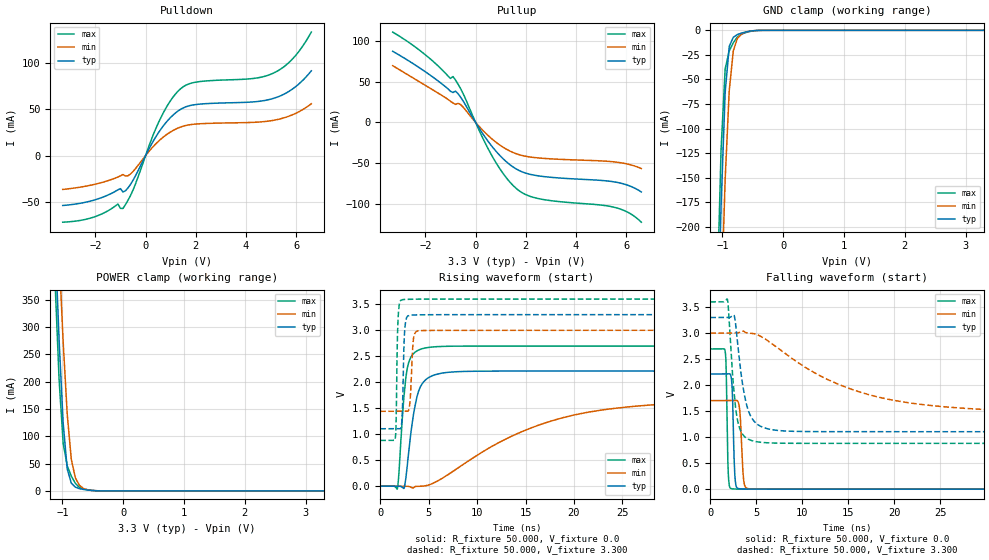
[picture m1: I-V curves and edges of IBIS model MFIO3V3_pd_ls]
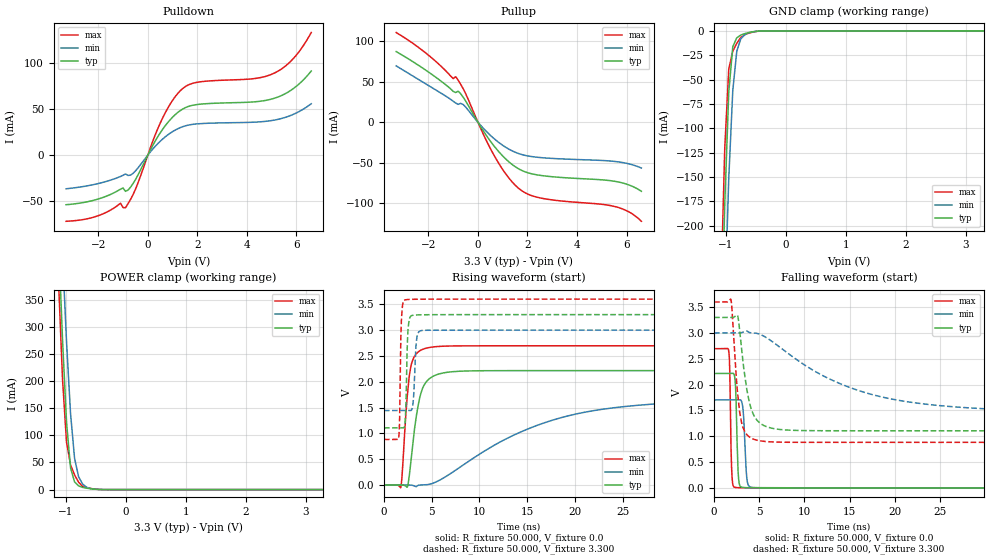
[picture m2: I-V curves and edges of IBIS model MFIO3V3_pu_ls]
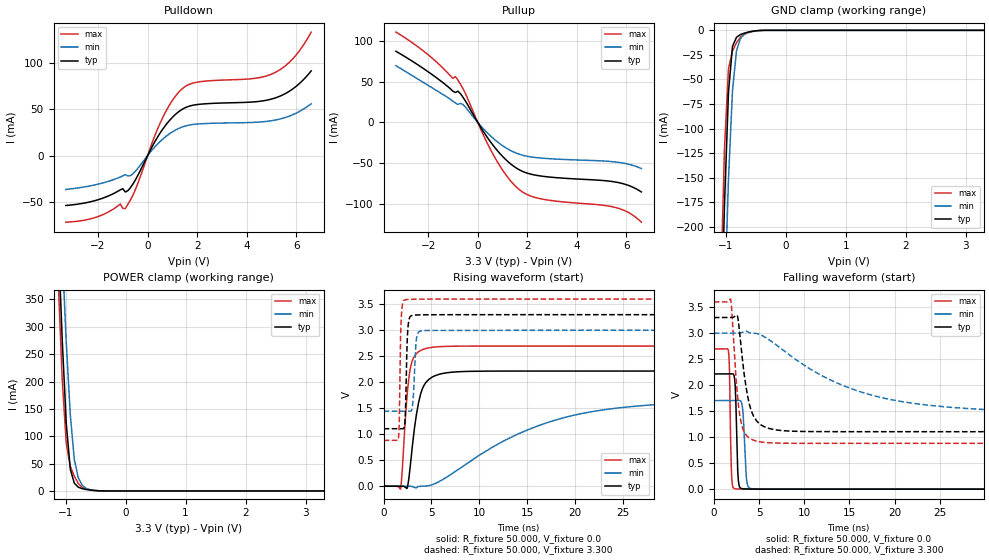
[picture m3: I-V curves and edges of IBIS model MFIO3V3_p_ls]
| IBIS file lpc55s0x_jbd64.ibs
[IBIS Ver]   5.0
[File name]   lpc55s0x_jbd64.ibs
[File Rev]   1.0
[Date]   August 08,2020
[Notes]   Rev History
|   1.0  initial release
[Disclaimer]   The model given below represents a 64-pin package.
[Copyright]   Copyright NXP 2020
[Component] lpc55s0x
[Manufacturer] NXP
[Package]
|   typ   min   max
R_pkg   0.19617   0.1259   0.24257
L_pkg   3.452e-9   2.657e-9   4.299e-9
C_pkg   5.434e-13   4.645e-13   6.669e-13
[Pin]   Signal_name   model_name   R_pin   L_pin   C_pin
32   VBAT_DCDC   POWER   NA   NA   NA
33   VBAT_PMU   POWER   NA   NA   NA
9   VDDA   POWER   NA   NA   NA
8   VDDE   POWER   NA   NA   NA
16   VDDE   POWER   NA   NA   NA
28   VDDE   POWER   NA   NA   NA
43   VDDE   POWER   NA   NA   NA
56   VDDE   POWER   NA   NA   NA
24   VDD_PMU   POWER   NA   NA   NA
10   VREFP   POWER   NA   NA   NA
29   FB   NC   0.21382   3.234e-9   5.594e-13
31   LX   NC   0.1259   2.657e-9   6.669e-13
36   P0_0   gpio3v3   0.18104   3.304e-9   5.312e-13
2   P0_1   gpio3v3   0.20833   3.785e-9   5.955e-13
54   P0_2   gpio3v3   0.19647   3.418e-9   5.268e-13
55   P0_3   gpio3v3   0.2007   3.265e-9   5.08e-13
57   P0_4   gpio3v3   0.20065   3.267e-9   5.147e-13
58   P0_5   gpio3v3   0.20039   3.463e-9   5.189e-13
59   P0_6   gpio3v3   0.20514   3.553e-9   5.526e-13
1   P0_7   gpio3v3   0.22402   4.088e-9   5.574e-13
17   P0_8   gpio3v3   0.21685   3.93e-9   5.333e-13
37   P0_9   gpio3v3   0.17288   3.178e-9   5.157e-13
13   P0_10   gpio3v3   0.18436   3.37e-9   5.571e-13
6   P0_11   gpio3v3   0.17442   3.19e-9   5.137e-13
5   P0_12   gpio3v3   0.18127   3.344e-9   5.397e-13
46   P0_13   iicgpio3v3   0.18768   3.399e-9   5.469e-13
47   P0_14   iicgpio3v3   0.19847   3.574e-9   5.659e-13
14   P0_15   gpio3v3   0.19509   3.491e-9   5.923e-13
7   P0_16   gpio3v3   0.17362   2.955e-9   4.961e-13
38   P0_18   gpio3v3   0.16738   3.09e-9   4.89e-13
60   P0_19   gpio3v3   0.21213   3.67e-9   5.623e-13
48   P0_20   gpio3v3   0.20914   3.854e-9   5.212e-13
49   P0_21   gpio3v3   0.22547   4.105e-9   5.559e-13
51   P0_22   gpio3v3   0.20602   3.668e-9   5.785e-13
12   P0_23   gpio3v3   0.17829   3.098e-9   5.305e-13
45   P0_24   gpio3v3   0.17877   3.257e-9   5.192e-13
52   P0_25   gpio3v3   0.2005   3.571e-9   5.586e-13
40   P0_26   gpio3v3   0.16383   2.973e-9   4.854e-13
18   P0_27   gpio3v3   0.20727   3.705e-9   5.696e-13
44   P0_28   gpio3v3   0.17962   3.062e-9   4.989e-13
61   P0_29   gpio3v3   0.21833   3.792e-9   5.854e-13
63   P0_30   gpio3v3   0.24257   4.299e-9   6.149e-13
15   P0_31   gpio3v3   0.21237   3.493e-9   6.058e-13
4   P1_0   gpio3v3   0.19044   3.496e-9   5.532e-13
39   P1_1   gpio3v3   0.16532   3.035e-9   4.645e-13
41   P1_2   gpio3v3   0.16584   2.976e-9   4.885e-13
42   P1_3   gpio3v3   0.17391   2.979e-9   4.668e-13
64   P1_4   gpio3v3   0.21758   3.972e-9   5.207e-13
22   P1_5   gpio3v3   0.19606   3.418e-9   5.2e-13
3   P1_9   gpio3v3   0.20144   3.654e-9   5.698e-13
25   P1_10   gpio3v3   0.20199   3.169e-9   5.208e-13
62   P1_11   gpio3v3   0.22784   3.919e-9   6.247e-13
21   P1_21   gpio3v3   0.19848   3.493e-9   5.331e-13
26   P1_22   gpio3v3   0.19791   3.34e-9   5.122e-13
27   P1_23   gpio3v3   0.20351   3.333e-9   5.169e-13
50   P1_25   gpio3v3   0.21369   3.798e-9   6.012e-13
53   P1_29   gpio3v3   0.19707   3.477e-9   5.49e-13
23   RESETN   gpio3v3   0.19717   3.324e-9   5.017e-13
35   XTAL32K_N   NC   0.18989   3.359e-9   5.665e-13
34   XTAL32K_P   NC   0.2095   3.368e-9   5.834e-13
19   XTAL32M_N   NC   0.20829   3.687e-9   5.553e-13
20   XTAL32M_P   NC   0.202   3.586e-9   5.404e-13
65   VSS   GND   NA   NA   NA
11   VSSA   GND   NA   NA   NA
30   VSS_DCDC   GND   NA   NA   NA
|   Model Selector
[Model Selector] gpio3v3
MFIO3V3_pd_hs  EPUN=1 EPD=1 EHS=1
MFIO3V3_pd_ls  EPUN=1 EPD=1 EHS=0
MFIO3V3_pu_hs  EPUN=0 EPD=0 EHS=1
MFIO3V3_pu_ls  EPUN=0 EPD=0 EHS=0
MFIO3V3_p_hs  EPUN=1 EPD=0 EHS=1
MFIO3V3_p_ls  EPUN=1 EPD=0 EHS=0
MFIO3V3_r_hs  EPUN=0 EPD=1 EHS=1
MFIO3V3_r_ls  EPUN=0 EPD=1 EHS=0
[Model Selector] iicgpio3v3
IIC3V3_pd_hs  EGP=1 EPUN=1 EPD=1 EHS=1
IIC3V3_pd_ls  EGP=1 EPUN=1 EPD=1 EHS=0
IIC3V3_p_hs  EGP=1 EPUN=1 EPD=0 EHS=1
IIC3V3_p_ls  EGP=1 EPUN=1 EPD=0 EHS=0
IIC3V3_pu_hs  EGP=1 EPUN=0 EPD=0 EHS=1
IIC3V3_pu_ls  EGP=1 EPUN=0 EPD=0 EHS=0
IIC3V3_r_hs  EGP=1 EPUN=0 EPD=1 EHS=1
IIC3V3_r_ls  EGP=1 EPUN=0 EPD=1 EHS=0
IIC3V3_pd_iic_hs  EGP=0 ECS=0 EPUN=1 EPD=1
IIC3V3_p_iic_hs  EGP=0 ECS=0 EPUN=1 EPD=0
IIC3V3_pu_iic_hs  EGP=0 ECS=0 EPUN=0 EPD=0
IIC3V3_r_iic_hs  EGP=0 ECS=0 EPUN=0 EPD=1
IIC3V3_pd_iic_pu_hs  EGP=0 ECS=1 EPUN=1 EPD=1  SSEL=1
IIC3V3_p_iic_pu_hs  EGP=0 ECS=1 EPUN=1 EPD=0  SSEL=1
IIC3V3_pu_iic_pu_hs  EGP=0 ECS=1 EPUN=0 EPD=0  SSEL=1
IIC3V3_r_iic_pu_hs  EGP=0 ECS=1 EPUN=0 EPD=1  SSEL=1
| Models and submodels in the file (24): MFIO3V3_pd_hs (I/O), MFIO3V3_pd_ls (I/O), MFIO3V3_pu_hs (I/O), MFIO3V3_pu_ls (I/O), MFIO3V3_p_hs (I/O), MFIO3V3_p_ls (I/O), MFIO3V3_r_hs (I/O), MFIO3V3_r_ls (I/O), IIC3V3_pd_hs (I/O), IIC3V3_pd_ls (I/O), IIC3V3_p_hs (I/O), IIC3V3_p_ls (I/O), IIC3V3_pu_hs (I/O), IIC3V3_pu_ls (I/O), IIC3V3_r_hs (I/O), IIC3V3_r_ls (I/O), IIC3V3_pd_iic_hs (I/O_open_drain), IIC3V3_p_iic_hs (I/O_open_drain), IIC3V3_pu_iic_hs (I/O_open_drain), IIC3V3_r_iic_hs (I/O_open_drain), IIC3V3_pd_iic_pu_hs (I/O_open_drain), IIC3V3_p_iic_pu_hs (I/O_open_drain), IIC3V3_pu_iic_pu_hs (I/O_open_drain), IIC3V3_r_iic_pu_hs (I/O_open_drain)
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|   Model MFIO3V3_pd_ls
[Model] MFIO3V3_pd_ls
Model_type I/O
Polarity   Non-Inverting
Enable   Active-Low
Vinl =  0.990V
Vinh =  2.310V
Vmeas =  1.650V
Cref =  0.0F
Rref =  100.000
Vref =  0.0V
C_comp   1.906pF   1.877pF   1.925pF
C_comp_pullup   1.141pF   1.113pF   1.145pF
C_comp_pulldown   0.641pF   0.601pF   0.647pF
[Model Spec]
Vinh   2.310V   2.100V   2.520V
Vinl   0.990V   0.900V   1.080V
Vmeas   1.650V   1.500V   1.800V
Vref   0.0V   0.0V   0.0V
Cref   0.0F   0.0F   0.0F
Rref   100.000   100.000   100.000
[Temperature Range]   25.000   0.125k   -40.000
[Voltage Range]   3.300V   3.000V   3.600V
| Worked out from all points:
|   slope of the pulldown table from 0 to 0.495 V, typ, clamps not added: 20.7 ohm
|   slope of the pullup table from 0 to 0.495 V, typ, clamps not added: 21.4 ohm
|   GND clamp passes 1 mA (typ) near -0.56 V on its own axis
|   POWER clamp passes 1 mA (typ) near -0.53 V on its own axis
|   rising waveform, R_fixture 50.000, V_fixture 0.0: 20-80 % time 1.05ns typ, 11.9ns min, 670ps max; typ from 0 V to 2.21 V
|   rising waveform, R_fixture 50.000, V_fixture 3.300: 20-80 % time 176ps typ, 234ps min, 146ps max; typ from 1.1 V to 3.3 V
|   falling waveform, R_fixture 50.000, V_fixture 0.0: 20-80 % time 203ps typ, 279ps min, 162ps max; typ from 2.21 V to 0 V
|   falling waveform, R_fixture 50.000, V_fixture 3.300: 20-80 % time 1.13ns typ, 11.2ns min, 744ps max; typ from 3.3 V to 1.1 V
[Pulldown]
|Voltage   I(typ)   I(min)   I(max)
-3.3V     -53.7mA    -36.43mA   -71.67mA
-2.1V     -48.29mA   -31.37mA   -66.51mA
-1.1V     -36.82mA   -23.05mA   -52.1mA
-900mV    -39.2mA    -20.39mA   -56.91mA
-600mV    -30.96mA   -19.83mA   -42.97mA
600mV     28.07mA    17.5mA     40.4mA
1V        41.17mA    25.53mA    59.41mA
1.4V      49.87mA    30.79mA    72.04mA
2V        54.93mA    33.94mA    79.03mA
5V        60.84mA    37.53mA    87.68mA
5.9V      72.62mA    44.52mA    105.4mA
6.6V      91.19mA    55.78mA    132.9mA
[Pullup]
|Voltage   I(typ)   I(min)   I(max)
-3.3V     87.16mA    69.54mA    110.7mA
-2.1V     64.12mA    47.22mA    85.31mA
-1V       38.1mA     25.85mA    53.88mA
-900mV    36.64mA    23.75mA    56.16mA
-800mV    38.25mA    22.02mA    51.93mA
-600mV    31.06mA    21.93mA    41.58mA
700mV     -31.25mA   -21.55mA   -43.56mA
1.2V      -47.6mA    -32.42mA   -66.97mA
1.7V      -58.52mA   -39.3mA    -83.05mA
2.6V      -66.01mA   -43.88mA   -94.06mA
5.6V      -73.4mA    -48.74mA   -104.7mA
6.6V      -85.32mA   -56.6mA    -122.4mA
[GND_clamp]
|Voltage   I(typ)   I(min)   I(max)
-3.3V     -7.222A    -7.177A    -7.278A
-1.089V   -337.1mA   -440.8mA   -274.1mA
-1.022V   -178.2mA   -284.2mA   -121mA
-955mV    -63.05mA   -151.6mA   -39.25mA
-888mV    -16.33mA   -61.34mA   -20.9mA
-821mV    -7.066mA   -20.84mA   -12.66mA
-754mV    -4.265mA   -8.157mA   -6.693mA
-687mV    -2.794mA   -3.896mA   -3.841mA
-620mV    -1.725mA   -1.894mA   -2.339mA
-419mV    -112.4uA   -138.2uA   -135uA
3.3V      0A         0A         0A
[POWER_clamp]
|Voltage   I(typ)   I(min)   I(max)
-3.3V     8.016A     7.986A     8.074A
-1.122V   463.8mA    614.4mA    385mA
-1.055V   276.3mA    435mA      203.9mA
-988mV    124.1mA    272.4mA    87.22mA
-921mV    40.03mA    140.2mA    45.68mA
-854mV    14.24mA    57.83mA    27.12mA
-787mV    6.921mA    23.8mA     13.77mA
-720mV    4.141mA    10.27mA    6.207mA
-653mV    2.682mA    4.42mA     3.699mA
-586mV    1.616mA    1.919mA    2.191mA
-452mV    346.9uA    411.9uA    422.9uA
3.3V      0A         0A         0A
[Ramp]
| variable   typ   min   max
dV/dt_r   1.328/1.048n   1.021/11.887n   1.617/0.670n
dV/dt_f   1.317/1.132n   0.935/11.171n   1.631/0.743n
R_load = 50.000
[Rising Waveform]
R_fixture= 50.000
V_fixture= 0.0
V_fixture_min= 0.0
V_fixture_max= 0.0
|time   V(typ)   V(min)   V(max)
0s        11.38nV    124.8nV    46.5nV
1.76ns    11.77uV    -379.4nV   -52.39mV
1.89ns    124.5uV    -254.1nV   156mV
2.47ns    -34.09mV   65.71uV    1.767V
2.93ns    642.6mV    -4.824mV   2.378V
3.75ns    1.693V     -3.224mV   2.598V
4.9ns     2.078V     17.79mV    2.667V
15.38ns   2.214V     1.106V     2.695V
25.84ns   2.214V     1.529V     2.695V
100ns     2.214V     1.702V     2.695V
[Rising Waveform]
R_fixture= 50.000
V_fixture= 3.300
V_fixture_min= 3.000
V_fixture_max= 3.600
|time   V(typ)   V(min)   V(max)
0s        1.105V     1.44V      880.4mV
1.55ns    1.105V     1.44V      919.2mV
1.85ns    1.105V     1.44V      3.271V
2.2ns     1.184V     1.44V      3.582V
2.34ns    1.855V     1.44V      3.589V
2.64ns    3.192V     1.44V      3.594V
3.07ns    3.287V     1.621V     3.596V
3.43ns    3.293V     2.839V     3.597V
4.06ns    3.296V     2.992V     3.598V
100ns     3.299V     2.999V     3.599V
[Falling Waveform]
R_fixture= 50.000
V_fixture= 0.0
V_fixture_min= 0.0
V_fixture_max= 0.0
|time   V(typ)   V(min)   V(max)
0s        2.214V     1.703V     2.695V
1.63ns    2.214V     1.703V     2.64V
1.73ns    2.214V     1.703V     2.3V
1.97ns    2.214V     1.703V     263mV
2.38ns    1.941V     1.702V     7.184mV
2.7ns     199.7mV    1.703V     3.012mV
3.2ns     7.193mV    1.527V     1.541mV
3.63ns    2.938mV    178.8mV    1.008mV
4.26ns    1.462mV    6.421mV    552.8uV
100ns     15.88nV    209.7nV    49.27nV
[Falling Waveform]
R_fixture= 50.000
V_fixture= 3.300
V_fixture_min= 3.000
V_fixture_max= 3.600
|time   V(typ)   V(min)   V(max)
0s        3.299V     2.999V     3.599V
1.87ns    3.299V     2.999V     3.646V
2.6ns     3.336V     2.999V     1.836V
3.1ns     2.603V     3.009V     1.222V
3.85ns    1.693V     3.011V     992.4mV
4.41ns    1.398V     2.998V     939.4mV
5.16ns    1.242V     2.965V     908.2mV
14.39ns   1.105V     1.984V     880.4mV
25.09ns   1.105V     1.589V     880.4mV
100ns     1.105V     1.44V      880.4mV
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|   Model MFIO3V3_pu_ls
[Model] MFIO3V3_pu_ls
Model_type I/O
Polarity   Non-Inverting
Enable   Active-Low
Vinl =  0.990V
Vinh =  2.310V
Vmeas =  1.650V
Cref =  0.0F
Rref =  100.000
Vref =  0.0V
C_comp   1.906pF   1.877pF   1.925pF
C_comp_pullup   1.139pF   1.112pF   1.144pF
C_comp_pulldown   0.643pF   0.602pF   0.649pF
[Model Spec]
Vinh   2.310V   2.100V   2.520V
Vinl   0.990V   0.900V   1.080V
Vmeas   1.650V   1.500V   1.800V
Vref   0.0V   0.0V   0.0V
Cref   0.0F   0.0F   0.0F
Rref   100.000   100.000   100.000
[Temperature Range]   25.000   0.125k   -40.000
[Voltage Range]   3.300V   3.000V   3.600V
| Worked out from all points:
|   slope of the pulldown table from 0 to 0.495 V, typ, clamps not added: 20.7 ohm
|   slope of the pullup table from 0 to 0.495 V, typ, clamps not added: 21.4 ohm
|   GND clamp passes 1 mA (typ) near -0.55 V on its own axis
|   POWER clamp passes 1 mA (typ) near -0.54 V on its own axis
|   rising waveform, R_fixture 50.000, V_fixture 0.0: 20-80 % time 1.05ns typ, 11.9ns min, 674ps max; typ from 0.001 V to 2.21 V
|   rising waveform, R_fixture 50.000, V_fixture 3.300: 20-80 % time 179ps typ, 230ps min, 146ps max; typ from 1.11 V to 3.3 V
|   falling waveform, R_fixture 50.000, V_fixture 0.0: 20-80 % time 203ps typ, 278ps min, 162ps max; typ from 2.21 V to 0.001 V
|   falling waveform, R_fixture 50.000, V_fixture 3.300: 20-80 % time 1.14ns typ, 11.2ns min, 744ps max; typ from 3.3 V to 1.11 V
[Pulldown]
|Voltage   I(typ)   I(min)   I(max)
-3.3V     -53.7mA    -36.43mA   -71.67mA
-2.1V     -48.29mA   -31.37mA   -66.51mA
-1.1V     -36.82mA   -23.05mA   -52.1mA
-900mV    -39.2mA    -20.39mA   -56.91mA
-600mV    -30.96mA   -19.83mA   -42.97mA
600mV     28.07mA    17.5mA     40.4mA
1V        41.17mA    25.53mA    59.41mA
1.4V      49.87mA    30.79mA    72.04mA
2V        54.93mA    33.94mA    79.03mA
5V        60.84mA    37.53mA    87.68mA
5.9V      72.62mA    44.52mA    105.4mA
6.6V      91.19mA    55.78mA    132.9mA
[Pullup]
|Voltage   I(typ)   I(min)   I(max)
-3.3V     87.16mA    69.54mA    110.7mA
-2.1V     64.12mA    47.22mA    85.31mA
-1V       38.1mA     25.85mA    53.88mA
-900mV    36.64mA    23.75mA    56.16mA
-800mV    38.25mA    22.02mA    51.93mA
-600mV    31.06mA    21.93mA    41.58mA
700mV     -31.25mA   -21.55mA   -43.56mA
1.2V      -47.6mA    -32.42mA   -66.97mA
1.7V      -58.52mA   -39.3mA    -83.05mA
2.6V      -66.01mA   -43.88mA   -94.06mA
5.6V      -73.4mA    -48.74mA   -104.7mA
6.6V      -85.32mA   -56.6mA    -122.4mA
[GND_clamp]
|Voltage   I(typ)   I(min)   I(max)
-3.3V     -7.222A    -7.177A    -7.278A
-1.089V   -337.2mA   -440.9mA   -274.2mA
-1.022V   -178.3mA   -284.2mA   -121.1mA
-955mV    -63.12mA   -151.7mA   -39.33mA
-888mV    -16.39mA   -61.39mA   -20.98mA
-821mV    -7.132mA   -20.89mA   -12.74mA
-754mV    -4.331mA   -8.209mA   -6.777mA
-687mV    -2.86mA    -3.948mA   -3.925mA
-620mV    -1.791mA   -1.946mA   -2.423mA
-419mV    -178.1uA   -190.3uA   -219.1uA
3.3V      0A         0A         0A
[POWER_clamp]
|Voltage   I(typ)   I(min)   I(max)
-3.3V     8.016A     7.986A     8.074A
-1.122V   463.7mA    614.3mA    385mA
-1.055V   276.3mA    434.9mA    203.9mA
-988mV    124mA      272.3mA    87.13mA
-921mV    39.96mA    140.1mA    45.6mA
-854mV    14.17mA    57.77mA    27.03mA
-787mV    6.855mA    23.75mA    13.68mA
-720mV    4.075mA    10.22mA    6.123mA
-653mV    2.616mA    4.368mA    3.615mA
-586mV    1.55mA     1.867mA    2.107mA
-452mV    281.1uA    359.9uA    338.7uA
3.3V      0A         0A         0A
[Ramp]
| variable   typ   min   max
dV/dt_r   1.329/1.048n   1.022/11.881n   1.617/0.670n
dV/dt_f   1.316/1.133n   0.935/11.179n   1.631/0.744n
R_load = 50.000
[Rising Waveform]
R_fixture= 50.000
V_fixture= 0.0
V_fixture_min= 0.0
V_fixture_max= 0.0
|time   V(typ)   V(min)   V(max)
0s        869.8uV    949.2uV    842.8uV
1.76ns    883.1uV    948.8uV    -50.04mV
1.91ns    1.009mV    949.1uV    208mV
2.46ns    -36.02mV   1.012mV    1.752V
2.89ns    574.4mV    -2.122mV   2.352V
3.71ns    1.664V     -1.354mV   2.595V
4.93ns    2.083V     22.11mV    2.669V
15.41ns   2.215V     1.111V     2.696V
25.89ns   2.215V     1.532V     2.696V
100ns     2.215V     1.704V     2.696V
[Rising Waveform]
R_fixture= 50.000
V_fixture= 3.300
V_fixture_min= 3.000
V_fixture_max= 3.600
|time   V(typ)   V(min)   V(max)
0s        1.106V     1.442V     881.7mV
1.55ns    1.106V     1.442V     920.7mV
1.83ns    1.106V     1.442V     3.201V
2.2ns     1.19V      1.442V     3.584V
2.36ns    2.014V     1.442V     3.591V
2.67ns    3.219V     1.441V     3.595V
3.05ns    3.288V     1.591V     3.597V
3.47ns    3.295V     2.885V     3.598V
4.05ns    3.297V     2.994V     3.599V
100ns     3.3V       3V         3.6V
[Falling Waveform]
R_fixture= 50.000
V_fixture= 0.0
V_fixture_min= 0.0
V_fixture_max= 0.0
|time   V(typ)   V(min)   V(max)
0s        2.215V     1.704V     2.696V
1.63ns    2.215V     1.704V     2.641V
1.73ns    2.215V     1.704V     2.3V
1.97ns    2.216V     1.704V     265.9mV
2.37ns    1.988V     1.704V     8.752mV
2.68ns    252.6mV    1.704V     4.211mV
3.22ns    8.138mV    1.493V     2.448mV
3.64ns    3.966mV    165.1mV    1.883mV
4.28ns    2.4mV      8.68mV     1.408mV
100ns     869.8uV    949.4uV    842.8uV
[Falling Waveform]
R_fixture= 50.000
V_fixture= 3.300
V_fixture_min= 3.000
V_fixture_max= 3.600
|time   V(typ)   V(min)   V(max)
0s        3.3V       3V         3.6V
1.88ns    3.3V       3V         3.639V
2.61ns    3.334V     3V         1.817V
3.06ns    2.664V     3.008V     1.251V
3.83ns    1.711V     3.015V     996.5mV
4.37ns    1.414V     3.001V     943.5mV
5.06ns    1.258V     2.975V     912.3mV
14.38ns   1.106V     1.987V     881.7mV
25.08ns   1.106V     1.591V     881.7mV
100ns     1.106V     1.442V     881.7mV
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|   Model MFIO3V3_p_ls
[Model] MFIO3V3_p_ls
Model_type I/O
Polarity   Non-Inverting
Enable   Active-Low
Vinl =  0.990V
Vinh =  2.310V
Vmeas =  1.650V
Cref =  0.0F
Rref =  100.000
Vref =  0.0V
C_comp   1.906pF   1.877pF   1.925pF
C_comp_pullup   1.140pF   1.112pF   1.144pF
C_comp_pulldown   0.642pF   0.602pF   0.649pF
[Model Spec]
Vinh   2.310V   2.100V   2.520V
Vinl   0.990V   0.900V   1.080V
Vmeas   1.650V   1.500V   1.800V
Vref   0.0V   0.0V   0.0V
Cref   0.0F   0.0F   0.0F
Rref   100.000   100.000   100.000
[Temperature Range]   25.000   0.125k   -40.000
[Voltage Range]   3.300V   3.000V   3.600V
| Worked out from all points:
|   slope of the pulldown table from 0 to 0.495 V, typ, clamps not added: 20.7 ohm
|   slope of the pullup table from 0 to 0.495 V, typ, clamps not added: 21.4 ohm
|   GND clamp passes 1 mA (typ) near -0.56 V on its own axis
|   POWER clamp passes 1 mA (typ) near -0.54 V on its own axis
|   rising waveform, R_fixture 50.000, V_fixture 0.0: 20-80 % time 1.05ns typ, 11.9ns min, 670ps max; typ from 0 V to 2.21 V
|   rising waveform, R_fixture 50.000, V_fixture 3.300: 20-80 % time 177ps typ, 237ps min, 147ps max; typ from 1.1 V to 3.3 V
|   falling waveform, R_fixture 50.000, V_fixture 0.0: 20-80 % time 203ps typ, 282ps min, 162ps max; typ from 2.21 V to 0 V
|   falling waveform, R_fixture 50.000, V_fixture 3.300: 20-80 % time 1.14ns typ, 11.2ns min, 740ps max; typ from 3.3 V to 1.1 V
[Pulldown]
|Voltage   I(typ)   I(min)   I(max)
-3.3V     -53.7mA    -36.43mA   -71.67mA
-2.1V     -48.29mA   -31.37mA   -66.51mA
-1.1V     -36.82mA   -23.05mA   -52.1mA
-900mV    -39.2mA    -20.39mA   -56.91mA
-600mV    -30.96mA   -19.83mA   -42.97mA
600mV     28.07mA    17.5mA     40.4mA
1V        41.17mA    25.53mA    59.41mA
1.4V      49.87mA    30.79mA    72.04mA
2V        54.93mA    33.94mA    79.03mA
5V        60.84mA    37.53mA    87.68mA
5.9V      72.62mA    44.52mA    105.4mA
6.6V      91.19mA    55.78mA    132.9mA
[Pullup]
|Voltage   I(typ)   I(min)   I(max)
-3.3V     87.16mA    69.54mA    110.7mA
-2.1V     64.12mA    47.22mA    85.31mA
-1V       38.1mA     25.85mA    53.88mA
-900mV    36.64mA    23.75mA    56.16mA
-800mV    38.25mA    22.02mA    51.93mA
-600mV    31.06mA    21.93mA    41.58mA
700mV     -31.25mA   -21.55mA   -43.56mA
1.2V      -47.6mA    -32.42mA   -66.97mA
1.7V      -58.52mA   -39.3mA    -83.05mA
2.6V      -66.01mA   -43.88mA   -94.06mA
5.6V      -73.4mA    -48.74mA   -104.7mA
6.6V      -85.32mA   -56.6mA    -122.4mA
[GND_clamp]
|Voltage   I(typ)   I(min)   I(max)
-3.3V     -7.222A    -7.177A    -7.278A
-1.089V   -337.1mA   -440.8mA   -274.1mA
-1.022V   -178.2mA   -284.2mA   -121mA
-955mV    -63.04mA   -151.6mA   -39.24mA
-888mV    -16.32mA   -61.33mA   -20.89mA
-821mV    -7.057mA   -20.83mA   -12.64mA
-754mV    -4.256mA   -8.15mA    -6.682mA
-687mV    -2.785mA   -3.888mA   -3.83mA
-620mV    -1.717mA   -1.887mA   -2.329mA
-419mV    -104.8uA   -131.8uA   -126uA
3.3V      0A         0A         0A
[POWER_clamp]
|Voltage   I(typ)   I(min)   I(max)
-3.3V     8.016A     7.986A     8.074A
-1.122V   463.7mA    614.3mA    384.9mA
-1.055V   276.2mA    434.9mA    203.8mA
-988mV    124mA      272.3mA    87.12mA
-921mV    39.95mA    140.1mA    45.59mA
-854mV    14.16mA    57.77mA    27.02mA
-787mV    6.846mA    23.74mA    13.67mA
-720mV    4.066mA    10.21mA    6.113mA
-653mV    2.607mA    4.361mA    3.605mA
-586mV    1.542mA    1.86mA     2.097mA
-452mV    273.4uA    353.7uA    329.6uA
3.3V      0A         0A         0A
[Ramp]
| variable   typ   min   max
dV/dt_r   1.329/1.049n   1.022/11.884n   1.618/0.670n
dV/dt_f   1.317/1.134n   0.935/11.178n   1.632/0.744n
R_load = 50.000
[Rising Waveform]
R_fixture= 50.000
V_fixture= 0.0
V_fixture_min= 0.0
V_fixture_max= 0.0
|time   V(typ)   V(min)   V(max)
0s        11.91nV    127.2nV    48.18nV
1.76ns    14.07uV    -353.2nV   -52.48mV
1.9ns     130.3uV    -106.1nV   185.6mV
2.46ns    -38.99mV   62.57uV    1.761V
2.93ns    644.9mV    -4.797mV   2.378V
3.65ns    1.606V     -5.408mV   2.586V
4.94ns    2.084V     20.24mV    2.669V
15.63ns   2.215V     1.125V     2.696V
25.83ns   2.215V     1.53V      2.696V
100ns     2.215V     1.703V     2.696V
[Rising Waveform]
R_fixture= 50.000
V_fixture= 3.300
V_fixture_min= 3.000
V_fixture_max= 3.600
|time   V(typ)   V(min)   V(max)
0s        1.105V     1.441V     880.7mV
1.55ns    1.105V     1.441V     919.6mV
1.84ns    1.105V     1.441V     3.233V
2.22ns    1.224V     1.441V     3.584V
2.37ns    2.139V     1.441V     3.59V
2.68ns    3.224V     1.44V      3.594V
3.06ns    3.287V     1.603V     3.596V
3.45ns    3.294V     2.861V     3.598V
4.07ns    3.297V     2.993V     3.599V
100ns     3.3V       3V         3.6V
[Falling Waveform]
R_fixture= 50.000
V_fixture= 0.0
V_fixture_min= 0.0
V_fixture_max= 0.0
|time   V(typ)   V(min)   V(max)
0s        2.215V     1.703V     2.696V
1.62ns    2.215V     1.703V     2.651V
1.73ns    2.215V     1.703V     2.303V
1.97ns    2.215V     1.703V     265.7mV
2.37ns    1.981V     1.703V     8.251mV
2.69ns    225.2mV    1.704V     3.621mV
3.22ns    7.595mV    1.492V     1.863mV
3.64ns    3.369mV    166.1mV    1.261mV
4.27ns    1.779mV    7.484mV    732uV
100ns     16.41nV    212.2nV    50.94nV
[Falling Waveform]
R_fixture= 50.000
V_fixture= 3.300
V_fixture_min= 3.000
V_fixture_max= 3.600
|time   V(typ)   V(min)   V(max)
0s        3.3V       3V         3.6V
1.88ns    3.3V       3V         3.641V
2.61ns    3.334V     3V         1.821V
3.08ns    2.642V     3.009V     1.24V
3.83ns    1.711V     3.015V     995.8mV
4.38ns    1.41V      3.001V     942.3mV
5.17ns    1.242V     2.968V     908.5mV
14.42ns   1.105V     1.984V     880.8mV
25.12ns   1.105V     1.59V      880.7mV
100ns     1.105V     1.441V     880.7mV
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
